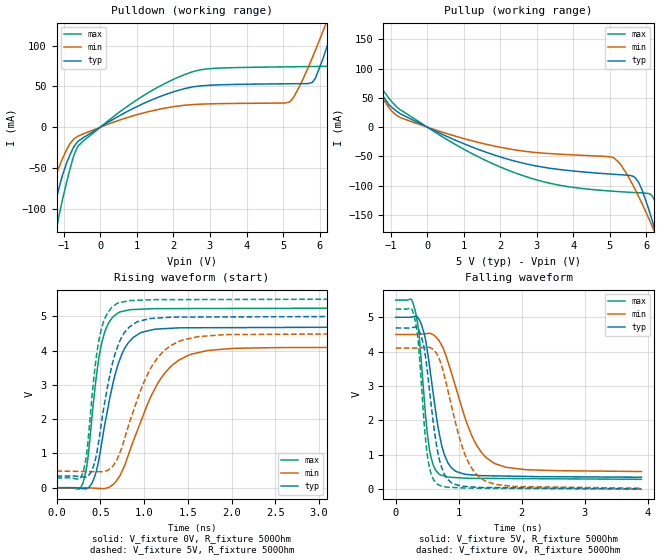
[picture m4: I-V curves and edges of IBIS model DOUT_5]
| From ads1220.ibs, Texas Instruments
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|   DOUT_5 Model
[Model]   DOUT_5
Model_type   3-state
Polarity   Non-Inverting
Vmeas = 2.5
Vref = 2.5
Cref = 15pF
Rref = 500
|   typ   min   max
|   (nom PVT)   (Fast PVT)   (slow PVT)
C_comp   2.718p   2.271p   3.185p
|C_comp (ON state)   2.856p   2.391p   3.337p
|C_comp (OFF state)   2.718p   2.271p   3.185p
| Where   nom PVT is  Nominal Process, 5V, 27C
|   Fast PVT is Strong Process, 5.5V, -40C
|   Slow PVT is Weak Process, 4.5V, 125C
[Voltage Range]   5   4.5   5.5
[Temperature Range]   27   125   -40
[Pullup Reference]   5   4.5   5.5
[Pulldown Reference]   0   0   0
[Power Clamp Reference]   5   4.5   5.5
[GND Clamp Reference]   0   0   0
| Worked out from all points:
|   slope of the pulldown table from 0 to 0.75 V, typ, clamps not added: 38.5 ohm
|   slope of the pullup table from 0 to 0.75 V, typ, clamps not added: 34.6 ohm
|   falling waveform, V_fixture 5V, R_fixture 500Ohm: 20-80 % time 231ps typ, 445ps min, 150ps max; typ from 5 V to 0.349 V
|   rising waveform, V_fixture 0V, R_fixture 500Ohm: 20-80 % time 233ps typ, 416ps min, 148ps max; typ from 0 V to 4.68 V
|   rising waveform, V_fixture 5V, R_fixture 500Ohm: 20-80 % time 214ps typ, 369ps min, 139ps max; typ from 0.34 V to 5 V
|   falling waveform, V_fixture 0V, R_fixture 500Ohm: 20-80 % time 203ps typ, 366ps min, 136ps max; typ from 4.69 V to 0.009 V
[Pulldown]
|   Voltage   I(typ)   I(min)   I(max)
-5V       -984.7mA   -666.3mA   -1.34A
-1.835V   -225.5mA   -142.5mA   -320.3mA
-1.52V    -154.3mA   -97.92mA   -220.6mA
-1.25V    -96.93mA   -62.99mA   -138.7mA
-605mV    -17.19mA   -11mA      -22.85mA
2.32V     47.36mA    26.92mA    64.68mA
5.17V     53.16mA    30.73mA    73.97mA
5.8V      54.77mA    84.97mA    74.32mA
6.25V     105.4mA    135.3mA    74.76mA
6.415V    129.1mA    154.2mA    79.06mA
7.09V     229.8mA    232.8mA    195.3mA
10V       695.5mA    589.2mA    793.5mA
[Pullup]
|   Voltage   I(typ)   I(min)   I(max)
-5V       615.3mA    484.3mA    781.6mA
-2.36V    216.2mA    176.1mA    268.1mA
-2.195V   191.6mA    157.1mA    236.3mA
-1.97V    158.2mA    131.4mA    193.3mA
-965mV    33.47mA    26.93mA    42.93mA
820mV     -23.56mA   -16.29mA   -31.34mA
2.95V     -65.85mA   -43.15mA   -89.22mA
5.095V    -80.35mA   -52.09mA   -109.3mA
5.695V    -86.53mA   -106.8mA   -111.6mA
6.25V     -178.5mA   -182.4mA   -127.7mA
6.49V     -231.1mA   -218.4mA   -172.3mA
10V       -1.077A    -812.1mA   -1.299A
[Ramp]
R_load = 500
|   typ   min   max
dV/dt_r   2.81122/2.31953e-10   2.45779/4.13764e-10   3.14302/1.47295e-10
dV/dt_f   2.79077/2.30674e-10   2.39144/4.43892e-10   3.12731/1.49622e-10
[Falling Waveform]
V_fixture = 5V
V_fixture_min = 4.5V
V_fixture_max = 5.5V
R_fixture = 500Ohm
C_fixture = 0F
|   Time   V(typ)   V(min)   V(max)
0s        5V         4.5V       5.5V
301.3ps   5.024V     4.5V       5.249V
371.3ps   4.936V     4.502V     4.473V
529ps     3.685V     4.532V     1.238V
685.9ps   1.663V     4.323V     444.6mV
769.3ps   1.022V     4.02V      383.9mV
935.2ps   542.4mV    3.072V     340.2mV
1.236ns   412mV      1.445V     316.7mV
1.544ns   388.3mV    775.6mV    313.3mV
3.9ns     348.7mV    514.3mV    287.8mV
[Rising Waveform]
V_fixture = 0V
V_fixture_min = 0V
V_fixture_max = 0V
R_fixture = 500Ohm
C_fixture = 0F
|   Time   V(typ)   V(min)   V(max)
0s        4.594nV    7.392nV    3.899nV
301.3ps   -24.2mV    1.124mV    139.9mV
356.5ps   -8.175mV   -908.9uV   823.3mV
413.5ps   178.3mV    -9.035mV   2.296V
505.6ps   1.141V     -22.14mV   4.09V
706.2ps   3.619V     283.1mV    5.102V
873.5ps   4.375V     1.338V     5.194V
1.154ns   4.626V     3.031V     5.221V
1.5ns     4.662V     3.854V     5.223V
3.9ns     4.685V     4.096V     5.238V
[Rising Waveform]
V_fixture = 5V
V_fixture_min = 4.5V
V_fixture_max = 5.5V
R_fixture = 500Ohm
C_fixture = 0F
|   Time   V(typ)   V(min)   V(max)
0s        340.2mV    485.1mV    286.7mV
297.8ps   318.2mV    474.7mV    416.5mV
347ps     325.1mV    472.9mV    1.061V
404.3ps   504.9mV    470.9mV    2.651V
490.1ps   1.488V     467.9mV    4.375V
685.9ps   4.033V     801.1mV    5.363V
829.5ps   4.681V     1.868V     5.454V
1.064ns   4.93V      3.427V     5.479V
1.397ns   4.974V     4.265V     5.485V
3.9ns     4.998V     4.494V     5.5V
[Falling Waveform]
|Gnd
V_fixture = 0V
V_fixture_min = 0V
V_fixture_max = 0V
R_fixture = 500Ohm
C_fixture = 0F
|   Time   V(typ)   V(min)   V(max)
0s        4.688V     4.104V     5.239V
297.8ps   4.711V     4.103V     4.998V
362.6ps   4.642V     4.106V     4.19V
499.9ps   3.458V     4.126V     1.018V
565.1ps   2.423V     4.1V       425.1mV
658.7ps   1.172V     3.912V     150.9mV
819ps     296.5mV    2.942V     59.86mV
1.091ns   81.82mV    1.045V     34.35mV
1.397ns   50.88mV    262.5mV    28.41mV
3.9ns     8.998mV    28.15mV    1.283mV
